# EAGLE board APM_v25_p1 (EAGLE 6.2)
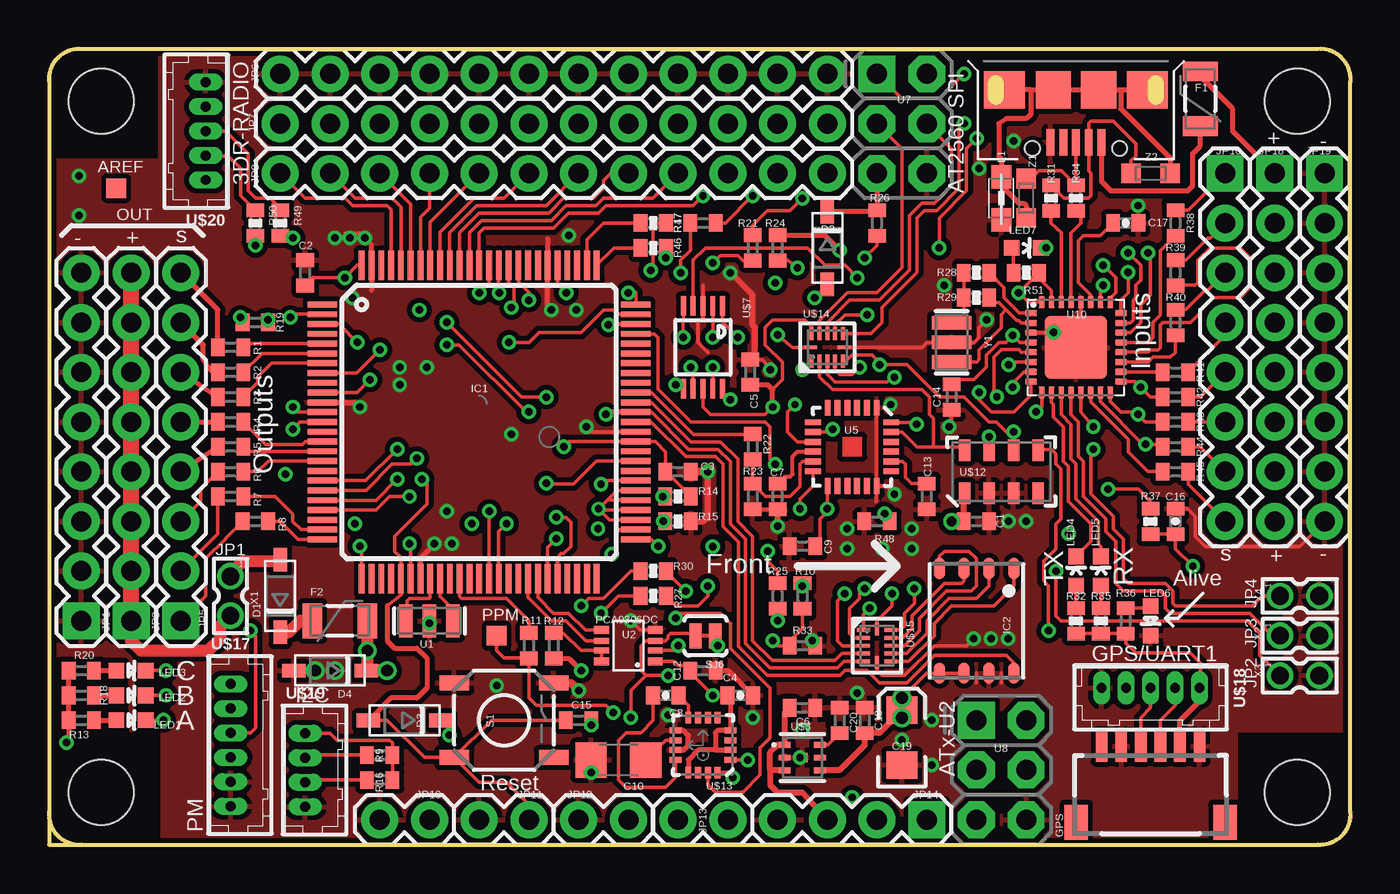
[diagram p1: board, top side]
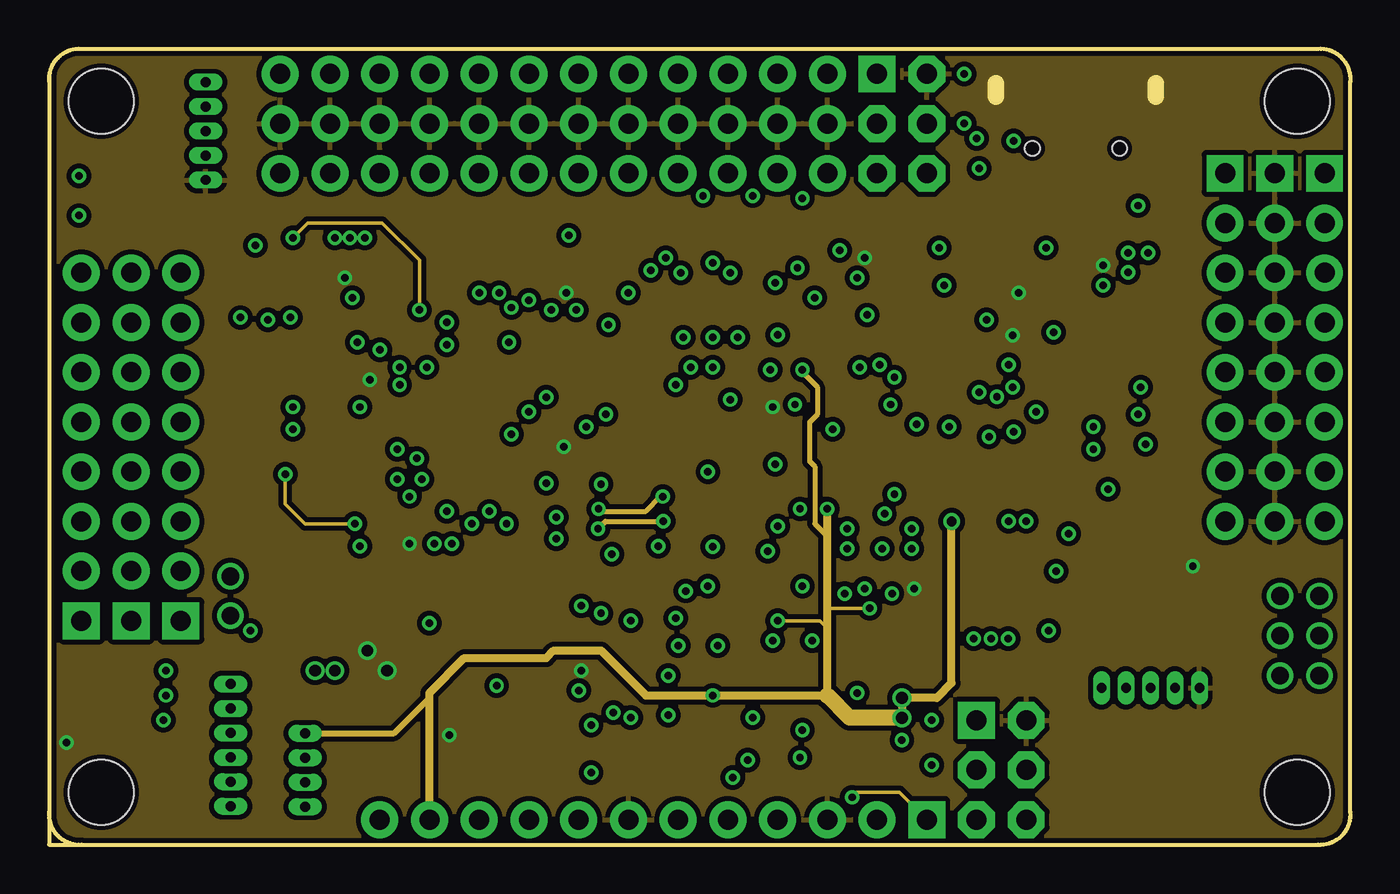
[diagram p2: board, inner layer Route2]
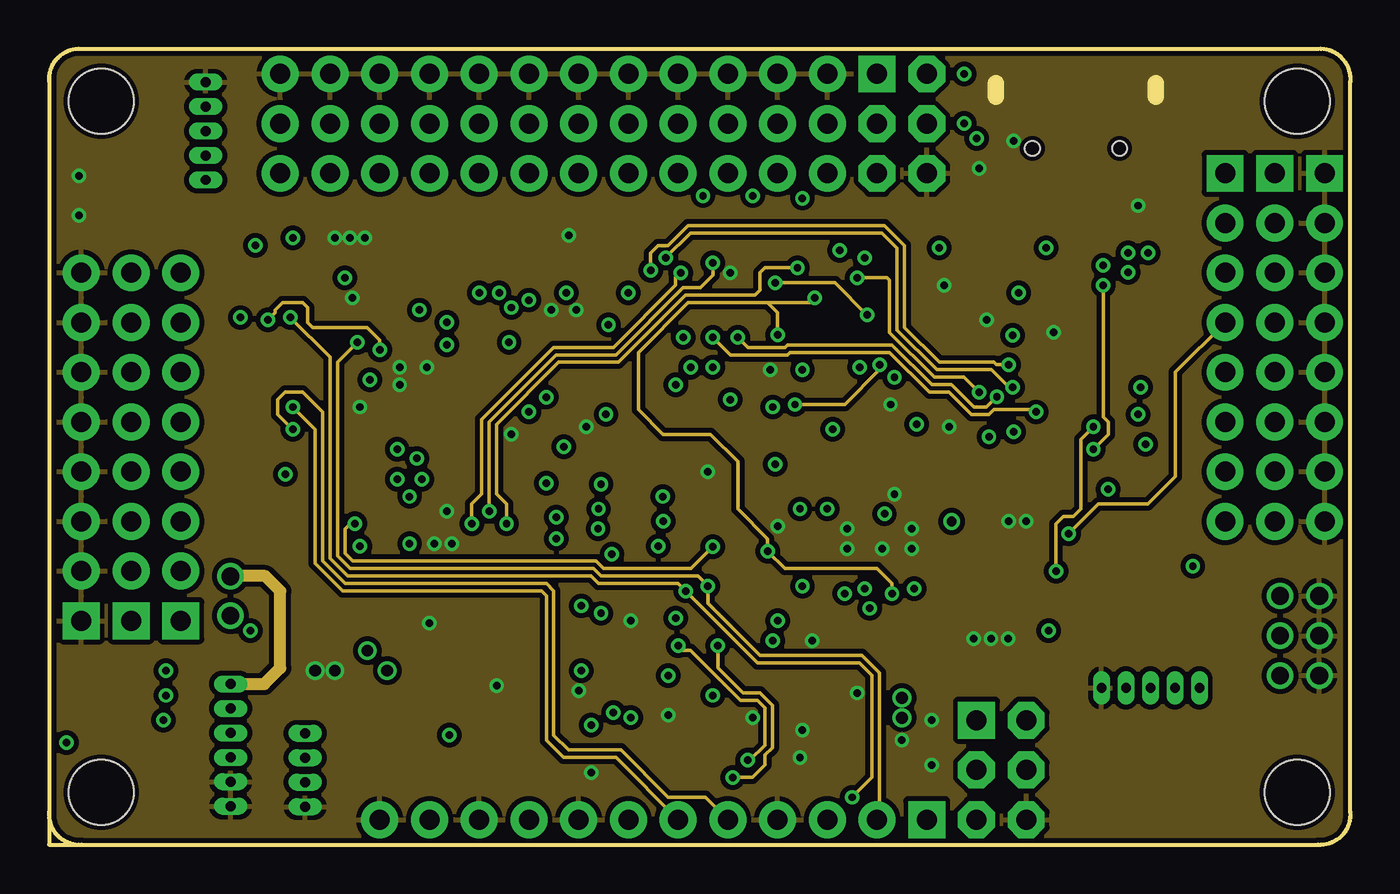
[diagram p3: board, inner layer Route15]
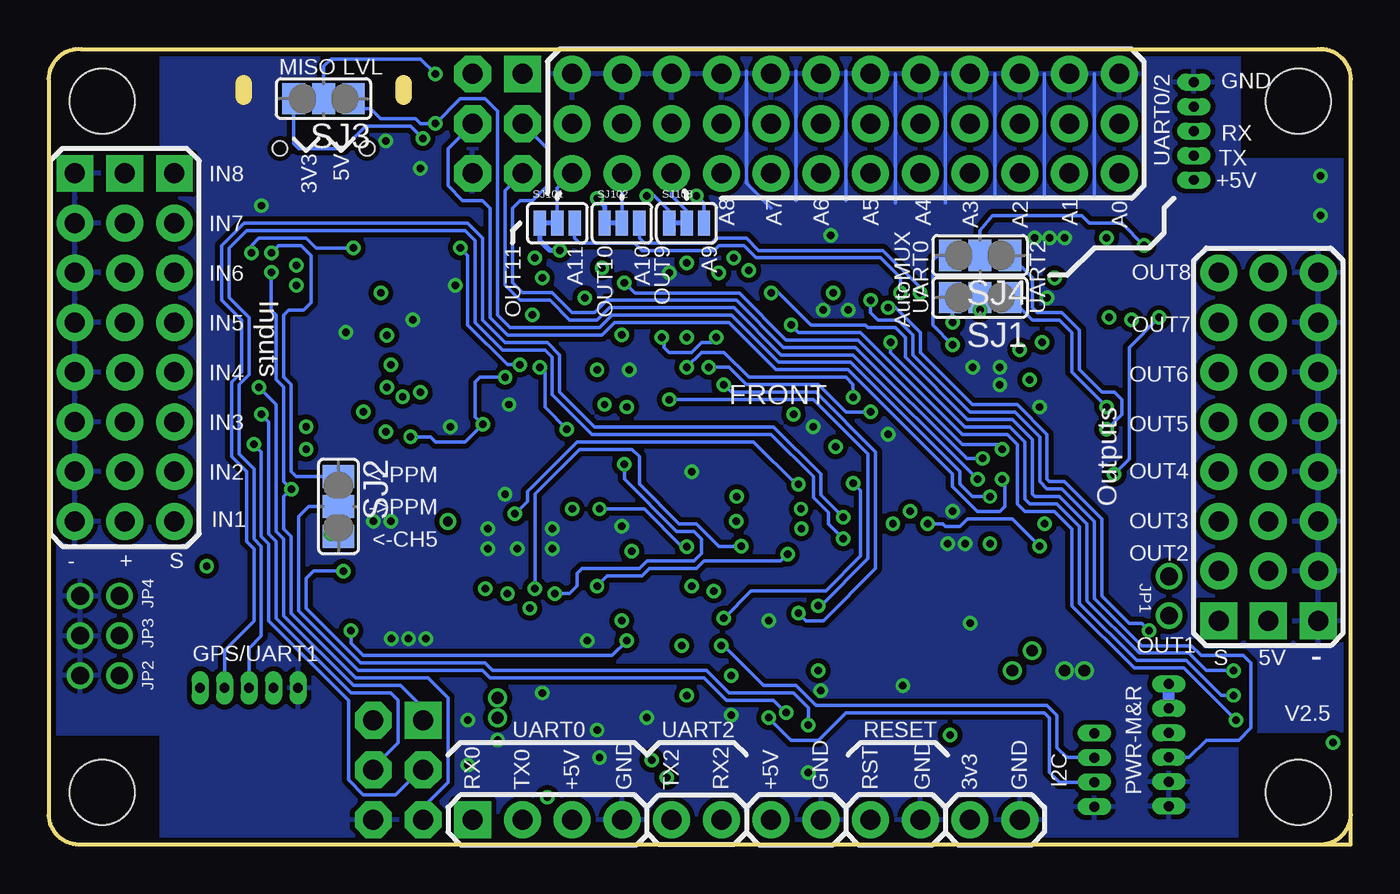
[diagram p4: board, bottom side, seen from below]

Size 66.48 x 40.65 mm. Coordinates in mm from the lower left corner, seen from the top.
Outline: 1.66,0 0,0 0,38.99
Outline: 1.66,0 64.83,0
Outline: 0,39.25 0,38.99
Outline: 1.4,40.64 64.83,40.64 arc-99 66.48,38.98 66.48,1.66 arc-99 64.82,0
Outline: 1.67,40.64 arc99 0,38.99
Outline: 0,1.67 arc99 1.66,0
Copper layers (1*2*15*16): Top 0.035mm / dielectric 0.5mm / Route2 0.035mm / dielectric 0.5mm / Route15 0.035mm / dielectric 0.5mm / Bottom 0.035mm
Design rules: minimum track width 7mil, minimum drill 10mil, track to track 7mil, track to pad 7mil, pad to pad 7mil, via to via 7mil, smd to smd 0mil, copper to edge 10mil, drill to drill 8mil, minimum pad ring 7mil, minimum via ring 7mil, stop-mask expansion 4mil, vias tented up to drill 25mil, thermal gap 10mil
Net classes: 0 default: width 0.178 mm, drill 0.381 mm, clearance 0.178 mm

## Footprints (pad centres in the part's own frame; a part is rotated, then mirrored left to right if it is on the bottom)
C0402 = smd 0.7 x 0.9: 1 -0.65,0; 2 0.65,0
0402-CAP = smd 0.7 x 0.9: 1 -0.65,0; 2 0.65,0
1206 = smd 1.6 x 1.8: 1 -1.4,0; 2 1.4,0
EIA3216 = smd 1.4 x 1.6: A 1.4,0; C -1.4,0
SOD-123 = smd 1.2 x 0.7: A 1.85,0; C -1.85,0
PTC-1206 = smd 1 x 1.8: 1 -1.4,0; 2 1.4,0
SM06B-SRSS-TB = smd 0.6 x 1.55: 1 -2.5,2.975; 2 -1.5,2.975; 3 -0.5,2.975; 4 0.5,2.975; 5 1.5,2.975; 6 2.5,2.975 | smd 1.2 x 1.8: FIT@1 -3.8,-0.9; FIT@2 3.8,-0.9
TQFP100 = smd 1.5 x 0.3: 1 -8,6; 2 -8,5.5; 3 -8,5; 4 -8,4.5; 5 -8,4; 6 -8,3.5; 7 -8,3; 8 -8,2.5; 9 -8,2; 10 -8,1.5; 11 -8,1; 12 -8,0.5; 13 -8,0; 14 -8,-0.5; 15 -8,-1; 16 -8,-1.5; 17 -8,-2; 18 -8,-2.5; 19 -8,-3; 20 -8,-3.5; 21 -8,-4; 22 -8,-4.5; 23 -8,-5; 24 -8,-5.5; 25 -8,-6; 51 8,-6; 52 8,-5.5; 53 8,-5; 54 8,-4.5; 55 8,-4; 56 8,-3.5; 57 8,-3; 58 8,-2.5; 59 8,-2; 60 8,-1.5; 61 8,-1; 62 8,-0.5; 63 8,0; 64 8,0.5; 65 8,1; 66 8,1.5; 67 8,2; 68 8,2.5; 69 8,3; 70 8,3.5; 71 8,4; 72 8,4.5; 73 8,5; 74 8,5.5; 75 8,6 | smd 0.3 x 1.5: 26 -6,-8; 27 -5.5,-8; 28 -5,-8; 29 -4.5,-8; 30 -4,-8; 31 -3.5,-8; 32 -3,-8; 33 -2.5,-8; 34 -2,-8; 35 -1.5,-8; 36 -1,-8; 37 -0.5,-8; 38 0,-8; 39 0.5,-8; 40 1,-8; 41 1.5,-8; 42 2,-8; 43 2.5,-8; 44 3,-8; 45 3.5,-8; 46 4,-8; 47 4.5,-8; 48 5,-8; 49 5.5,-8; 50 6,-8; 76 6,8; 77 5.5,8; 78 5,8; 79 4.5,8; 80 4,8; 81 3.5,8; 82 3,8; 83 2.5,8; 84 2,8; 85 1.5,8; 86 1,8; 87 0.5,8; 88 0,8; 89 -0.5,8; 90 -1,8; 91 -1.5,8; 92 -2,8; 93 -2.5,8; 94 -3,8; 95 -3.5,8; 96 -4,8; 97 -4.5,8; 98 -5,8; 99 -5.5,8; 100 -6,8
VDFN-8-NO-BOTTOM-PAD = smd 1.1 x 0.6: 1 -2.675,1.905; 2 -2.675,0.635; 3 -2.675,-0.635; 4 -2.675,-1.905; 5 2.675,-1.905; 6 2.675,-0.635; 7 2.675,0.635; 8 2.675,1.905
1X08 = drill 1.016 pad 1.88 square: 1 0,0 | drill 1.016 pad 1.88: 2 2.54,0; 3 5.08,0; 4 7.62,0; 5 10.16,0; 6 12.7,0; 7 15.24,0; 8 17.78,0
1X12 = drill 1.016 pad 1.88: 1 0,0; 2 2.54,0; 3 5.08,0; 4 7.62,0; 5 10.16,0; 6 12.7,0; 7 15.24,0; 8 17.78,0; 9 20.32,0; 10 22.86,0; 11 25.4,0; 12 27.94,0
1X02 = drill 1.016 pad 1.88: 1 0,0; 2 2.54,0
1X04 = drill 1.016 pad 1.88 square: 1 0,0 | drill 1.016 pad 1.88: 2 2.54,0; 3 5.08,0; 4 7.62,0
0805 = smd 1.2 x 1: 1 -1.1,0; 2 1.1,0
LED-0603 = smd 0.8 x 0.8: A 0,-0.75; C 0,0.75
0402-RES = smd 0.7 x 0.9: 1 -0.65,0; 2 0.65,0
TACTILE_SWITCH_SMD = smd 1.524 x 0.762: 1 -2.54,1.905; 2 2.54,1.905; 3 -2.54,-1.905; 4 2.54,-1.905
SJ_2 = smd 1.168 x 1.6: 1 -1.524,0; 2 0,0; 3 1.524,0
SJ_2S-TRACE = smd 0.635 x 1.27: 1 -0.508,0; 2 0.508,0
SJ_3 = smd 0.635 x 1.27: 1 -0.889,0; 2 0,0; 3 0.889,0
TP10SQ = smd 1 x 1: TP 0,0
RESONATOR-SMD = smd 0.7 x 1.7: 1 -1.2,0; 2 0,0; 3 1.2,0
VSSOP8 = smd 0.75 x 0.4: 1 -1.375,0.8; 4 -1.375,-0.8; 5 1.375,-0.8; 8 1.375,0.8 | smd 0.75 x 0.3: 2 -1.375,0.25; 3 -1.375,-0.25; 6 1.375,-0.25; 7 1.375,0.25
QFN-24 = smd 0.8 x 0.3: 1 -2,1.25; 2 -2,0.75; 3 -2,0.25; 4 -2,-0.25; 5 -2,-0.75; 6 -2,-1.25; 13 2,-1.25; 14 2,-0.75; 15 2,-0.25; 16 2,0.25; 17 2,0.75; 18 2,1.25 | smd 0.3 x 0.8: 7 -1.25,-2; 8 -0.75,-2; 9 -0.25,-2; 10 0.25,-2; 11 0.75,-2; 12 1.25,-2; 19 1.25,2; 20 0.75,2; 21 0.25,2; 22 -0.25,2; 23 -0.75,2; 24 -1.25,2
2X3-NS = drill 1.016 pad 1.88 square: 1 -2.54,-1.27 | drill 1.016 pad 1.88 octagon: 2 -2.54,1.27; 3 0,-1.27; 4 0,1.27; 5 2.54,-1.27; 6 2.54,1.27
MOLEX_MICRO_USB_AB_BOTTOM_MOUNT = smd 0.4 x 1.35: 1 1.3,-4.125; 2 0.65,-4.125; 3 0,-4.125; 4 -0.65,-4.125; 5 -1.3,-4.125 | smd 2.1 x 1.9: GND1 3.65,-1.452; GND4 -3.65,-1.452 | smd 1.8 x 1.9: GND2 1.151,-1.452; GND3 -1.149,-1.452 | hole 0.75: -2.225,-4.45; 2.225,-4.45
QFN32 = smd 0.6 x 0.3: 1 -2.3,1.75; 2 -2.3,1.25; 3 -2.3,0.75; 4 -2.3,0.25; 5 -2.3,-0.25; 6 -2.3,-0.75; 7 -2.3,-1.25; 8 -2.3,-1.75; 17 2.3,-1.75; 18 2.3,-1.25; 19 2.3,-0.75; 20 2.3,-0.25; 21 2.3,0.25; 22 2.3,0.75; 23 2.3,1.25; 24 2.3,1.75 | smd 0.3 x 0.6: 9 -1.75,-2.3; 10 -1.25,-2.3; 11 -0.75,-2.3; 12 -0.25,-2.3; 13 0.25,-2.3; 14 0.75,-2.3; 15 1.25,-2.3; 16 1.75,-2.3; 25 1.75,2.3; 26 1.25,2.3; 27 0.75,2.3; 28 0.25,2.3; 29 -0.25,2.3; 30 -0.75,2.3; 31 -1.25,2.3; 32 -1.75,2.3 | smd 3.2 x 3.2: EXP 0,0
STAND-OFF = hole 3.302: 0,0
MLF-6 = smd 0.6 x 0.3: 1 -0.9,0.65; 2 -0.9,0; 3 -0.9,-0.65; 4 0.9,-0.65; 5 0.9,0; 6 0.9,0.65 | smd 0.5 x 0.5: 7 0,0
MSOP10 = smd 0.25 x 1: 1 -1,-2.113; 2 -0.5,-2.113; 3 0,-2.113; 4 0.5,-2.113; 5 1,-2.113; 6 1,2.113; 7 0.5,2.113; 8 0,2.113; 9 -0.5,2.113; 10 -1,2.113
MS5611-01BA = smd 1.1 x 0.6: 1 -1.1,1.875; 2 -1.1,0.625; 3 -1.1,-0.625; 4 -1.1,-1.875; 5 1.1,-1.875; 6 1.1,-0.625; 7 1.1,0.625; 8 1.1,1.875
LPCC16 = smd 0.6 x 0.3: 1 -1.4,0.75; 2 -1.4,0.25; 3 -1.4,-0.25; 4 -1.4,-0.75; 9 1.4,-0.75; 10 1.4,-0.25; 11 1.4,0.25; 12 1.4,0.75 | smd 0.3 x 0.6: 5 -0.75,-1.4; 6 -0.25,-1.4; 7 0.25,-1.4; 8 0.75,-1.4; 13 0.75,1.4; 14 0.25,1.4; 15 -0.25,1.4; 16 -0.75,1.4
UQFN-12 = smd 0.2 x 0.65: 1 -0.8,-0.7; 2 -0.4,-0.7; 3 0,-0.7; 4 0.4,-0.7; 5 0.8,-0.7; 7 0.8,0.7; 8 0.4,0.7; 9 0,0.7; 10 -0.4,0.7; 11 -0.8,0.7 | smd 0.65 x 0.2: 6 0.85,0; 12 -0.85,0
DF13-6P-1.25DSA = drill 0.5 pad 0.8 long: 1 -3.125,0; 2 -1.875,0; 3 -0.625,0; 4 0.625,0; 5 1.875,0; 6 3.125,0
DF13-5P-1.25DSA = drill 0.5 pad 0.8 long: 1 -2.5,0; 2 -1.25,0; 3 0,0; 4 1.25,0; 5 2.5,0
DF13-4P-1.25DSA = drill 0.5 pad 0.8 long: 1 -1.875,0; 2 -0.625,0; 3 0.625,0; 4 1.875,0
87758-0216 = drill 0.9 pad 1.27: 1 0,-1; 2 0,1
RESONATOR = smd 0.7 x 2: 1 -1,0; 2 0,0; 3 1,0
CT/CN0603 = smd 1 x 1: 1 -1,0; 2 1,0

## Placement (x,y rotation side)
C1  .1uF  [C0402]  47.38,16.51 180 top
C2  .1uF  [C0402]  13.09,29.21 90 top
C3  .1uF  [C0402]  32.14,19.05 0 top
C4  0.1uF  [0402-CAP]  35.31,7.62 0 top
C5  .1uF  [C0402]  35.82,24.13 270 top
C6  1uF  [C0402]  38.49,6.99 180 top
C7  .1uF  [C0402]  37.22,17.78 90 top
C8  0.22uF  [0402-CAP]  31.5,7.62 180 top
C9  .1uF  [C0402]  38.49,15.24 0 top
C10  4.7uF  [1206]  29.09,4.32 180 top
C12  .1uF  [C0402]  33.41,8.89 180 top
C13  .01uF  [C0402]  44.84,17.78 90 top
C14  .1uF  [C0402]  46.11,22.86 270 top
C15  .1uF  [C0402]  27.06,6.35 180 top
C16  .1uF  [0402-CAP]  57.54,16.51 90 top
C17  1uF  [0402-CAP]  55,31.75 0 top
C18  .01uF  [C0402]  41.66,6.35 270 top
C19  10uf  [EIA3216]  43.57,5.47 90 top
C20  470pF  [C0402]  40.39,6.35 270 top
D1  MBR120VLSFT1G  [SOD-123]  11.82,12.7 90 top
D2  MBR120VLSFT1G  [SOD-123]  39.76,30.48 270 top
D3  MBR120VLSFT1G  [SOD-123]  18.17,6.35 180 top
D4  MMSZ5233BT1G  [SOD-123]  14.36,8.89 180 top
F1  500mA  [PTC-1206]  58.81,38.1 90 top
F2  500mA  [PTC-1206]  14.86,11.43 0 top
GPS  SM06B-SRSS-TB  [SM06B-SRSS-TB]  56.27,2.04 0 top
IC1  ATMEGA2560-16AU  [TQFP100]  21.98,21.59 0 top
IC2  AT45DB161D-MU  [VDFN-8-NO-BOTTOM-PAD]  47.38,11.43 270 top
JP1  GND  [1X08]  1.66,11.43 90 top
JP3  5V  [1X08]  4.2,11.43 90 top
JP5  OUT PWM  [1X08]  6.74,11.43 90 top
JP6  GND  [1X12]  11.82,39.37 0 top
JP7  5V  [1X12]  11.82,36.83 0 top
JP8  IO pins  [1X12]  11.82,34.29 0 top
JP10  3v3  [1X02]  19.44,1.27 180 top
JP11  RST  [1X02]  24.52,1.27 180 top
JP12  VCC  [1X02]  27.06,1.27 0 top
JP13  UART2  [1X02]  34.68,1.27 180 top
JP14  UART0  [1X04]  44.84,1.27 180 top
JP16  IN PWM  [1X08]  60.08,34.29 270 top
JP18  5V  [1X08]  62.62,34.29 270 top
JP19  GND  [1X08]  65.16,34.29 270 top
L1  BLM21  [0805]  48.65,33.02 90 top
LED1  RED  [LED-0603]  4.2,6.35 270 top
LED2  YELLOW  [LED-0603]  4.2,7.62 270 top
LED3  BLUE  [LED-0603]  4.2,8.89 270 top
LED4  ORANGE  [LED-0603]  52.46,13.97 0 top
LED5  ORANGE  [LED-0603]  53.73,13.97 0 top
LED6  GRN  [LED-0603]  56.27,11.43 180 top
LED7  RED  [LED-0603]  49.92,30.48 270 top
R1  220  [C0402]  9.28,25.4 0 top
R2  220  [C0402]  9.28,24.13 0 top
R3  220  [C0402]  9.28,22.86 0 top
R4  220  [C0402]  9.28,21.59 0 top
R5  220  [C0402]  9.28,20.32 0 top
R6  220  [C0402]  9.28,19.05 0 top
R7  220  [C0402]  9.28,17.78 0 top
R8  220  [C0402]  10.55,16.51 0 top
R9  2.2k  [C0402]  16.9,4.58 0 top
R10  4.7K  [C0402]  38.49,12.7 90 top
R11  1K  [C0402]  24.52,10.16 270 top
R12  200k  [C0402]  25.79,10.16 270 top
R13  1k  [C0402]  1.66,6.35 180 top
R14  10K  [0402-RES]  32.14,17.78 180 top
R15  10K  [0402-RES]  32.14,16.51 180 top
R16  2.2k  [C0402]  16.9,3.31 0 top
R17  1k  [C0402]  33.41,31.75 0 top
R18  1k  [C0402]  1.66,7.62 180 top
R19  220  [C0402]  10.55,26.67 0 top
R20  1k  [C0402]  1.66,8.89 180 top
R21  1k  [C0402]  35.95,30.48 90 top
R22  4.7K  [C0402]  35.95,20.32 90 top
R23  10k  [C0402]  35.95,17.78 270 top
R24  1k  [C0402]  37.22,30.48 90 top
R25  10k  [C0402]  37.22,12.7 90 top
R26  10k  [C0402]  42.3,31.75 270 top
R27  1k  [0402-RES]  30.87,12.7 180 top
R28  27  [0402-RES]  47.38,29.21 0 top
R29  1M  [0402-RES]  47.38,27.94 180 top
R30  1k  [0402-RES]  30.87,13.97 180 top
R31  22  [0402-RES]  51.19,33.02 90 top
R32  1k  [0402-RES]  52.46,11.43 90 top
R33  10k  [C0402]  38.49,10.16 0 top
R34  22  [0402-RES]  52.46,33.02 90 top
R35  1k  [0402-RES]  53.73,11.43 90 top
R36  1k  [C0402]  55,11.43 270 top
R37  10K  [0402-RES]  56.27,16.51 270 top
R38  220  [C0402]  57.54,31.75 270 top
R39  220  [C0402]  57.54,29.21 270 top
R40  220  [C0402]  57.54,26.67 270 top
R41  220  [C0402]  57.54,24.13 180 top
R42  220  [C0402]  57.54,22.86 180 top
R43  220  [C0402]  57.54,21.59 180 top
R44  220  [C0402]  57.54,20.32 180 top
R45  220  [C0402]  57.54,19.05 180 top
R46  1k  [0402-RES]  30.87,30.48 0 top
R47  1k  [0402-RES]  30.87,31.75 0 top
R48  10k  [C0402]  42.3,16.51 180 top
R49  1k  [0402-RES]  11.82,31.75 270 top
R50  1k  [0402-RES]  10.55,31.75 270 top
R51  1k  [0402-RES]  49.92,29.21 180 top
S1  [TACTILE_SWITCH_SMD]  23.25,6.35 0 top
SJ1  [SJ_2]  18.93,27.94 180 bottom
SJ2  [SJ_2]  51.69,17.28 270 bottom
SJ3  [SJ_2]  52.46,38.1 180 bottom
SJ4  [SJ_2]  18.93,30.1 180 bottom
SJ6  MAG  [SJ_2S-TRACE]  33.53,10.67 180 top
SJ101  [SJ_3]  40.52,31.75 0 bottom
SJ102  [SJ_3]  37.22,31.75 0 bottom
SJ103  [SJ_3]  33.91,31.75 0 bottom
TP1  TPSQTP10SQ  [TP10SQ]  3.43,33.53 0 top
TP2  TPSQTP10SQ  [TP10SQ]  22.86,10.67 0 top
U1  16MHZ  [RESONATOR-SMD]  19.44,11.43 0 top
U2  PCA9306DC  [VSSOP8]  29.6,10.16 180 top
U5  MPU-6000  [QFN-24]  41.03,20.32 270 top
U7  SPI_Mega  [2X3-NS]  43.57,36.83 270 top
U8  SPI_PPM  [2X3-NS]  48.65,3.81 270 top
U9  USB  [MOLEX_MICRO_USB_AB_BOTTOM_MOUNT]  52.46,40.01 0 top
U10  ATMEGA32U2-MU  [QFN32]  52.46,25.4 0 top
U$1  STAND-OFF  [STAND-OFF]  2.67,37.98 0 top
U$2  STAND-OFF  [STAND-OFF]  2.67,2.67 0 top
U$3  MIC5219-3V3  [MLF-6]  38.49,4.45 0 top
U$4  STAND-OFF  [STAND-OFF]  63.76,37.98 0 top
U$5  STAND-OFF  [STAND-OFF]  63.76,2.67 0 top
U$6  CREATIVE_COMMONS  [CREATIVE_COMMONS]  not placed on the board
U$7  TS5A23157  [MSOP10]  33.41,25.4 180 top
U$12  MS5611-01BA  [MS5611-01BA]  48.65,19.05 90 top
U$13  HMC5883L  [LPCC16]  33.41,5.08 180 top
U$14  TS  [UQFN-12]  39.76,25.4 0 top
U$15  QFN  [UQFN-12]  42.3,10.16 270 top
U$17  DF13-6P-1.25DSA  [DF13-6P-1.25DSA]  9.28,5.08 270 top
U$18  DF13-5P-1.25DSA  [DF13-5P-1.25DSA]  56.27,8.01 180 top
U$19  DF13-4P-1.25DSA  [DF13-4P-1.25DSA]  13.09,3.81 270 top
U$20  DF13-5P-1.25DSA  [DF13-5P-1.25DSA]  8.01,36.45 90 top
X1  ESC 5V EN  [87758-0216]  9.28,12.7 180 top
X2  PPM_PD6  [87758-0216]  63.89,10.67 270 top
X3  HWB  [87758-0216]  63.89,8.64 270 top
X4  PPM_PC4  [87758-0216]  63.89,12.7 270 top
Y1  16MHz  [RESONATOR]  46.11,25.66 90 top
Z1  PGB1010604  [CT/CN0603]  49.92,33.02 270 top
Z2  PGB1010604  [CT/CN0603]  56.27,34.29 0 top

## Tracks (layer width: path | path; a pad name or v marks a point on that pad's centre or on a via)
3.3V  (via drill 0.38, 0.5, 0.6)
  Top 0.178: U2.1 31.92,9.36 32.14,9.15 32.5,9.15 C12.2 32.76,8.78 v33.91,7.62 | U5.13 39.78,17.26 v39.76,17.15 | v39.76,17.15 39.76,17.02 39.37,16.64 39.37,15.5 39.11,15.23 C9.2 | v37.22,11.43 R25.1 | v39.76,17.15 39.74,17.15 | U$14.1 38.93,24.7 v38.49,24.26 | IC2.6 IC2.5 44.83,8.76 v43.57,7.5 | U$15.1 41.6,11.75 v41.91,12.07 | R16.2 R9.2 17.55,5.2 17.4,5.34 14.71,5.34 14.36,5.69 U$19.1
  Top 0.254: v33.91,7.62 C4.1 34.81,7.48 U$13.4 34.16,5.83 34.04,5.72 34.04,4.83 | 34.04,4.83 33.16,4.83 32.66,4.33 U$13.13 | 34.04,4.83 U$13.2
  Top 0.305: U$12.1 46.73,17.91 C1.2 | U$3.4 40.38,3.8 41.66,5.08 C18.2 42.41,5.7 43.18,6.48 v43.57,6.48
  Top 0.406: v43.57,6.48 C19.A | v46.11,16.51 C1.2
  Route2 0.178: v37.22,11.43 39.37,11.43 39.76,11.05 | v41.91,12.07 39.76,12.07
  Route2 0.254: v38.49,24.26 38.49,24.13 39.25,23.37 39.25,21.98 38.87,21.59 38.87,19.56 39.12,19.31 39.12,16.39 39.76,15.75
  Route2 0.305: U$19.1 17.63,5.69 19.44,7.5
  Route2 0.406: JP10.1 19.44,7.5 19.44,7.75 21.21,9.53 25.4,9.53 25.79,9.91 28.2,9.91 30.48,7.62 v33.91,7.62 39.76,7.62 39.76,11.05 39.76,12.07 39.76,15.75 v39.76,17.15 | v43.57,6.48 v43.57,7.5 45.34,7.5 46.11,8.26 v46.11,16.51
  Route2 0.813: v43.57,6.48 40.9,6.48 39.76,7.62
5V
  Top 0.254: 4.32,12.7 4.2,12.83
  Top 0.61: JP3.1 4.2,10.42 4.7,9.91 8.13,9.91 8.77,10.55 8.77,11.2 X1.2
  Top 0.813: JP3.1 4.2,12.83 JP3.2 JP3.3 JP3.4 JP3.5 JP3.6 JP3.7 JP3.8
#RST  (via drill 0.38)
  Top 0.178: U10.13 52.71,22.11 v53.34,21.34 | v51.44,13.97 51.44,11.69 51.69,11.43 61.22,11.43 61.85,10.8 61.85,9.67 X3.1
  Top 0.406: C15.1 27.71,6.12 v27.69,6.1
  Route15 0.178: v53.34,21.34 52.71,20.71 52.71,17.15 52.33,16.77 51.82,16.77 51.44,16.39 v51.44,13.97
  Bottom 0.178: v27.69,6.1 27.69,6.99 28.45,7.75 31.75,7.75 32.9,8.89 43.82,8.89 44.2,9.28 50.55,9.28 53.34,12.07 53.34,13.59 52.96,13.97 v51.44,13.97
CH1
  Top 0.178: R45.1 58.19,18.4 JP16.8
CH5  (via drill 0.38)
  Top 0.178: JP16.4 60.08,26.04 58.19,24.15 R41.1
  Route15 0.178: JP16.4 57.54,24.13 57.54,18.8 56.14,17.4 53.6,17.4 v52.07,15.88
  Bottom 0.178: SJ2.3 52.2,15.75 v52.07,15.88
CH8
  Top 0.178: JP16.1 58.19,32.4 R38.1
CS_DF
  Top 0.178: U$15.9 43.69,10.16 44.45,10.93 44.45,11.56 45.85,12.96 47.12,12.96 47.38,13.21 47.38,14.61 46.99,14.99 45.72,14.99 45.47,14.74 IC2.4
CS_MS5611  (via drill 0.38)
  Top 0.178: U$12.5 50.55,20.18 51.2,20.18 51.44,19.94 51.44,19.44 51.69,19.18 51.69,16.64 51.44,16.39 51.44,15.12 50.8,14.48 50.8,13.47 51.06,13.21 v51.06,10.93 | 38.5,12.07 R10.1 38.49,11.05 37.85,10.42 R33.1 37.22,10.16 v36.96,10.42
  Bottom 0.178: v51.06,10.93 51.06,10.29 50.42,9.66 37.72,9.66 v36.96,10.42
D+
  Top 0.178: Z1.1 50.15,34.02 50.55,34.42 51.71,34.42 R34.2 U9.3
D-
  Top 0.178: R31.2 51.84,33.02 53.09,33.02 53.22,33.15 53.22,34.29 53.11,34.41 U9.2 53.11,36.85 53.22,36.96 54.36,36.96 55.5,35.82 55.5,35.18 55.27,34.95 Z2.1
FSYNC
  Top 0.178: U5.11 38.5,19.57 38.36,19.44 38.36,18.29 37.85,17.78 36.6,17.78 R23.1 R22.1
GND  (via drill 0.38, 0.6)
  Top 0.178: IC1.62 27.69,21.09 v27.44,21.34 | U10.3 v51.32,26.15 | 51.95,25.91 51.71,26.15 v51.32,26.15 | 51.95,25.91 U10.EXP | v51.32,26.15 v51.31,26.17 | U1.2 v19.44,11.31 | U5.1 U5.18 42.77,18.32 v43.18,17.91 | R23.2 C7.1 | C16.2 58.16,17.16 58.55,16.77 58.55,15.75 59.06,15.24 63.89,15.24 JP19.8 | C5.1 36.44,24.78 v36.83,24.26 | U$7.3 33.41,26.93 33.15,26.67 33.15,25.66 33.66,25.15 | 16.48,30.65 v16.13,30.99 15.88,31.25 15.12,31.25 | C14.2 46.11,21.59 v45.98,21.34 | U2.4 30.19,10.96 v29.72,11.43 | U$15.6 42.3,8.89 42.55,8.64 43.69,8.64 45.22,10.16 46.87,10.16 47.25,10.55 | U$14.6 44.58,25.4 44.84,25.66 Y1.2 47.25,25.66 47.5,25.91 47.5,26.42 v47.88,26.8 47.76,26.67 | R33.2 39.14,10.28 v38.99,10.42 | U10.28 52.71,26.67 51.95,25.91 | 33.41,27.69 33.41,28.58 | 47.38,8.77 47.38,8.26 | 48.65,8.77 48.65,8.26 | 42.27,18.24 42.27,17.56 42.24,17.53
  Top 0.254: IC1.11 15.61,22.59 v15.88,22.36 | IC1.81 25.48,27.49 v25.66,27.31 | IC1.62 | 16.48,30.65 IC1.99 16.48,28.32 | C4.2 34.68,8.89 C12.1 | U$13.11 32.39,4.83 32.64,5.08 32.64,5.59 32.4,5.83 U$13.9 | IC1.32 18.98,14.66 v19.69,15.37 | IC1.81 25.48,30.94
  Top 0.305: C7.1 v37.22,16.26 | R15.1 33.41,16.51 33.66,16.77 v33.66,19.05 | v34.8,29.21 35.95,28.07 35.95,26.55 36.07,26.42 36.07,25.04 C5.1
  Top 0.406: C3.2 33.14,19.04 v33.66,19.05 | S1.2 26.67,8.26 v27.06,7.88
  Bottom 0.178: 13.09,33.02 13.09,39.37 | 15.63,33.02 15.63,39.37 | 18.17,33.02 18.17,39.37 | 20.71,32.77 20.71,39.37 | 23.25,32.77 23.25,39.37 | 25.79,32.9 25.79,39.5 | 28.33,32.9 28.33,39.5 | 30.87,39.5 30.87,33.79 29.6,32.52
  other vias: 19.31,24.39 22.86,8.13 23.63,20.96 47.5,34.55 45.72,28.58 17.91,24.39 17.91,23.5 20.32,17.02 15.5,27.94 27.69,3.69 45.09,4.07 1.53,32.14 1.53,34.17 45.09,6.35 49.03,16.51 43.57,5.34 38.36,4.45 31.63,6.61 35.95,6.48 38.49,5.85 41.28,7.75 49.28,35.95 55.63,32.64 13.59,8.89 14.61,8.89 49.92,16.51 44.07,16.13 44.07,15.12 42.55,15.12 40.77,15.12 40.77,16.13 42.98,22.48 15.37,30.99 14.61,30.99 20.58,15.37 26.93,27.31 26.55,31.12 48.11,10.52 49,10.52 47.22,10.52
  pour Top (isolate 0.254): 14.74,28.96 29.21,28.83 29.21,14.23 14.74,14.36
  pour Bottom (isolate 0.254): 5.72,40.64 60.71,40.64 60.71,35.06 70.24,35.06 70.24,5.72 60.71,5.72 60.71,0 5.85,0 5.85,5.85 0,5.85 0,34.93 5.72,34.93
  pour Route15 (isolate 0.254): 0,40.64 67.7,40.64 67.7,0 0,0
  pour Top (isolate 0.254): 0,34.93 5.72,34.93 5.72,40.64 60.71,40.64 60.71,35.06 71.51,35.06 71.51,5.85 60.58,5.85 60.58,0 5.85,0 5.85,5.85 0,5.85
HI  (via drill 0.38)
  Top 0.178: IC1.54 28.13,17.09 v28.07,17.15 | IC1.55 29.96,17.61 28.53,17.61 v28.07,17.15 | IC1.53 28.63,16.59 v28.07,17.15 | IC1.56 29.02,18.09 v28.07,17.15
  Top 0.254: v31.36,17.78 R14.2
  Route2 0.254: v31.36,17.78 31.25,17.78 30.48,17.02 28.2,17.02 v28.07,17.15
IN0
  Top 0.178: 53.21,22.62 U10.14 53.22,23.09 53.22,22.61 55.12,20.71 55.12,20.07 56.14,19.05 R45.2
IN4
  Top 0.178: U10.18 56.87,24.15 R41.2
IN5
  Top 0.178: R40.2 57.54,25.15 57.28,24.9 56.39,24.9 56.15,24.65 U10.19
IN6
  Top 0.178: 57.52,28.58 R39.2 57.55,28.58 58.55,28.58 58.68,28.71 58.68,29.85 59.31,30.48 60.84,30.48 61.35,29.98 61.35,28.45 60.84,27.94 59.44,27.94 58.81,27.31 58.81,27.18 58.3,26.67 56.9,26.67 56.77,26.55 56.77,25.4 56.65,25.28 56.27,25.28 56.14,25.15 U10.20
IN7
  Top 0.178: U10.21 56.13,25.65 56.39,25.91 56.39,26.67 56.77,27.06 56.77,30.34 R38.2
INT  (via drill 0.38)
  Top 0.178: v38.36,17.15 38.36,17.66 39.03,18.33 U5.12 | R19.1 9.9,26.82 v9.78,26.93
  Route2 0.178: v12.07,18.93 12.07,17.4 13.09,16.39 v15.63,16.39
  Route15 0.178: v33.91,15.23 32.79,14.1 28.33,14.1 27.94,14.48 15.5,14.48 15.12,14.86 15.12,16.13 15.37,16.39 v15.63,16.39
  Bottom 0.178: v38.36,17.15 36.07,17.15 34.17,15.24 v33.91,15.23 | v9.78,26.93 11.31,25.4 11.31,19.69 v12.07,18.93
JP_RX  (via drill 0.38)
  Top 0.178: v12.45,30.99 11.93,30.99 R49.2
  Route2 0.178: v18.93,27.31 18.93,29.85 17.02,31.75 13.21,31.75 v12.45,30.99
  Bottom 0.178: SJ1.2 v18.93,27.31
JP_TX  (via drill 0.38)
  Top 0.178: v10.55,30.61 R50.2
  Bottom 0.178: v10.55,30.61 11.69,31.75 13.34,31.75 13.72,32.14 18.29,32.14 18.93,31.37 SJ4.2
JP_VCC
  Top 0.406: 11.76,14.61 D1.A
  Top 0.61: X1.1 9.28,13.85 9.91,14.48 11.74,14.48 D1.A
  Route15 0.61: U$17.1 11,8.21 11.82,9.02 11.82,12.96 11.05,13.72 9.29,13.72 X1.1
  Bottom 0.61: U$17.2 U$17.1
LO  (via drill 0.38)
  Top 0.254: v31.37,16.51 R15.2
  Route2 0.254: v28.05,16.13 28.43,16.51 v31.37,16.51
MISO_3V3  (via drill 0.38)
  Top 0.178: 49.27,21.08 U$12.6 | v49.28,21.09 49.27,21.08 | U5.9 38.24,20.57 37.72,21.09 37.72,22.1 v38.1,22.48 | U$14.5 40.71,24.7 41.03,25.02 42.04,25.02 42.42,24.64 v42.42,24.52 43.82,24.52 45.47,22.86 46.74,22.86 48.01,21.59 48.39,21.59 48.91,21.08 49.27,21.08 | v45.47,30.48 45.47,32.01 46.87,33.41 46.87,35.56 v47.38,36.07
  Route15 0.178: v38.1,22.48 40.64,22.48 42.42,24.26 v42.42,24.52
  Bottom 0.178: v42.42,24.52 43.06,24.52 45.09,26.55 45.09,30.1 v45.47,30.48 | v47.38,36.07 48.01,36.71 50.3,36.71 51.44,35.56 53.73,35.56 53.98,35.82 SJ3.3
MOSI_3V3  (via drill 0.38)
  Top 0.178: U$12.7 48.02,20.82 v48.01,20.83 | U5.24 44.22,21.57 v44.33,21.47 | U$14.3 39.76,24.01 40.14,23.63 42.8,23.63 v43.18,23.88
  Bottom 0.178: v48.01,20.83 46.99,20.83 46.74,20.58 45.22,20.58 v44.33,21.47 44.71,21.85 44.71,23.63 44.45,23.88 v43.18,23.88
MOSI_DF
  Top 0.178: U$15.7 43.91,9.36 45.22,10.67 45.22,11.31 46.11,12.2 48.26,12.2 49.28,13.21 IC2.1
MUX_RX  (via drill 0.38)
  Top 0.178: U$7.9 v33.91,24.38 v33.91,24.39 | v25.4,22.86 24.13,22.86 v20.32,26.67
  Bottom 0.178: v33.91,24.39 33.15,25.15 32.01,25.15 30.74,23.88 25.79,23.88 25.4,23.5 v25.4,22.86 | v20.32,26.67 20.32,27.82 SJ1.3
MUX_TX  (via drill 0.38)
  Top 0.178: U$7.7 32.91,24.25 v32.77,24.39 | v24.52,22.1 24.39,22.1 20.96,25.53 v20.32,25.53
  Bottom 0.178: v32.77,24.39 31.75,24.39 30.87,23.5 27.18,23.5 25.79,22.1 v24.52,22.1 | v20.32,25.53 21.34,26.55 21.34,29.85 21.09,30.1 SJ4.3 19.05,30.1
N$1
  Top 0.178: R36.1 56.17,12.08 LED6.A
N$2
  Top 0.178: U5.20 43.6,19.57 43.74,19.44 43.74,18.75 44.05,18.44 C13.2
N$3
  Top 0.203: U5.10 38.24,20.07 37.98,19.82 37.98,18.93 37.85,18.8 37.59,18.8 C7.2
N$4
  Top 0.178: U$3.6 39.79,5.1 C20.2
N$5
  Top 0.61: D1.C 12.25,10.85 12.83,11.43 F2.1
N$7
  Top 0.178: U$13.10 31.5,5.33 C10.1
N$8
  Top 0.254: JP5.5 R4.1
N$9
  Top 0.254: JP5.6 R3.1
N$10
  Top 0.254: JP5.7 7.88,25.53 7.88,24.77 8.01,24.64 8.01,24.52 8.39,24.13 R2.1
N$11
  Top 0.254: R1.1 8.63,27.32 JP5.8
N$12
  Top 0.178: U2.8 U2.7 27.18,9.91 26.29,10.8 25.8,10.8 R12.1
N$13
  Top 0.254: JP5.4 R5.1
N$14
  Top 0.178: R6.1 8.63,19.04 7.75,18.17 7.75,17.53 JP5.3
N$15
  Top 0.178: R7.1 8.63,15.86 JP5.2
N$16
  Top 0.178: R8.1 9.02,15.64 9.02,15.63 8.01,14.61 8.01,12.7 JP5.1
N$17
  Bottom 0.178: 19.05,27.94 20.32,27.94
N$18
  Top 0.178: R51.2 49.27,30.38 LED7.A
N$19
  Top 0.178: JP16.2 59.31,30.99 59.19,30.99 58.06,29.86 R39.1
N$20
  Top 0.178: R40.1 58.06,27.32 59.06,28.33 59.19,28.33 JP16.3
N$21
  Bottom 0.178: 51.19,38.23 52.2,38.23
N$22
  Top 0.178: R42.1 58.81,22.86 JP16.5
N$23
  Top 0.178: R43.1 JP16.6
N$24
  Top 0.178: R44.1 58.81,20.32 JP16.7
N$25  (via drill 0.38)
  Top 0.178: U$13.16 34.68,3.68 v34.93,3.43 | v34.17,10.16 SJ6.1
  Route15 0.178: v34.93,3.43 35.95,3.43 36.58,4.07 36.58,4.58 36.96,4.96 36.96,7.12 36.33,7.75 35.44,7.75 34.17,9.02 v34.17,10.16
N$26
  Top 0.178: U$13.8 32.66,7.12 C8.1
N$27
  Top 0.178: C8.2 30.85,6.34 30.23,5.72 29.47,5.72 29.09,5.34 29.09,3.31 29.47,2.93 31.5,2.93 32.01,3.43 U$13.12
N$28
  Top 0.254: R13.1 LED1.A
N$29
  Top 0.178: LED5.A R35.2
N$30
  Top 0.178: LED4.A R32.2
N$31
  Top 0.254: R18.1 LED2.A
N$32  (via drill 0.38)
  Top 0.178: R30.2 29.72,13.97 28.33,12.58 27.56,12.58 v27.18,12.2 | U$7.10 34.41,23.1 v34.8,22.74
  Bottom 0.178: v27.18,12.2 27.06,12.2 24.64,14.61 24.64,19.94 27.44,22.74 v34.8,22.74
N$33  (via drill 0.38)
  Top 0.178: R27.2 29.09,12.7 v28.2,11.82 | U$7.6 32.41,23.39 32.37,23.39 32.26,23.5 v32.01,23.5
  Bottom 0.178: v28.2,11.82 27.82,11.43 26.93,11.43 24.26,14.1 24.26,20.07 27.31,23.12 31.63,23.12 v32.01,23.5
N$34
  Top 0.254: R20.1 LED3.A
N$36  (via drill 0.38)
  Top 0.178: R17.2 34.55,31.75 v35.95,33.15
  Bottom 0.178: v35.95,33.15 35.56,33.15 34.8,32.39 SJ103.1
N$38  (via drill 0.38)
  Top 0.254: R24.2 39.61,31.13 v40.39,30.36
  Bottom 0.254: v40.39,30.36 40.9,30.36 41.41,30.87 SJ101.1
N$39  (via drill 0.38)
  Top 0.178: R21.2 35.95,31.63 36.71,32.39 37.85,32.39 v38.49,33.02
  Bottom 0.254: v38.49,33.02 38.23,32.77 38.1,32.64 SJ102.1
N$40
  Bottom 0.254: 34.04,31.75 34.68,31.75
N$41
  Bottom 0.254: 37.34,31.75 37.98,31.75
N$42
  Bottom 0.254: 40.77,31.75 41.15,31.75
N$56
  Top 0.178: IC1.34 19.98,12.67 20.64,12.01 U1.3 20.58,11.49
N$89
  Top 0.178: IC1.33 19.48,12.62 19.44,12.58 18.42,12.58 18.29,12.45 18.29,11.49 U1.1
PA1
  Top 0.178: IC1.77 27.48,30.9 28.33,31.75 R47.1
PA2
  Top 0.178: R46.1 28.87,30.48 IC1.76
PA3  (via drill 0.38)
  Top 0.178: IC1.75 29.98,28.2 v29.6,28.2 | LED3.C v5.97,8.89
  Bottom 0.178: v29.6,28.2 29.21,28.2 27.56,26.55 24.77,26.55 24.64,26.42 23.25,26.42 22.74,25.91 22.74,24.9 19.56,21.72 17.28,21.72 16.26,20.71 16.26,17.91 16.13,17.78 14.86,17.78 13.47,16.39 13.47,12.45 10.8,9.78 8.26,9.78 7.37,8.89 v5.97,8.89
PA4  (via drill 0.38)
  Top 0.178: IC1.74 29.05,27.09 28.83,27.31 28.33,27.31 27.18,26.17 25.02,26.17 24.52,25.66 v23.5,25.66 | LED2.C v5.97,7.62
  Bottom 0.178: v23.5,25.66 23.5,25.15 19.69,21.34 17.4,21.34 16.64,20.58 16.64,17.66 16.39,17.4 14.99,17.4 13.85,16.26 13.85,12.32 10.93,9.4 8.39,9.4 6.61,7.62 v5.97,7.62
PA5  (via drill 0.38)
  Top 0.178: IC1.73 28.63,26.59 v28.58,26.55 | LED1.C v5.85,6.35
  Bottom 0.178: v28.58,26.55 28.2,26.17 25.02,26.17 19.82,20.96 17.53,20.96 17.02,20.45 17.02,17.4 16.64,17.02 15.12,17.02 14.23,16.13 14.23,12.2 11.05,9.02 8.51,9.02 v5.85,6.35
PA6  (via drill 0.38)
  Top 0.178: IC1.72 30.94,26.09 31.12,25.91 31.12,23.27 32.8,21.59 36.58,21.59 36.83,21.34 36.83,19.69 v37.09,19.44 | U$15.3 40.52,10.16 40.26,10.42 40.26,12.45 v40.64,12.83
  Bottom 0.178: v37.09,19.44 37.09,18.67 34.42,16.01 33.53,16.01 33.15,15.63 33.15,14.86 33.53,14.48 35.95,14.48 36.33,14.1 39.25,14.1 39.5,13.85 39.5,13.21 39.88,12.83 v40.64,12.83
PB0  (via drill 0.38)
  Top 0.178: IC1.19 16.18,18.59 v17.78,20.2 | U$14.8 40.16,26.57 40.64,27.06 v41.79,27.06
  Route15 0.178: v41.79,27.06 40.14,28.71 v37.09,28.71
  Bottom 0.178: v37.09,28.71 36.56,28.17 31.22,28.17 28.83,25.79 25.15,25.79 19.82,20.45 18.04,20.45 v17.78,20.2
PB1  (via drill 0.38)
  Top 0.178: IC1.20 16.19,18.09 17.53,19.44 18.51,19.44 v18.8,19.73 | U$14.10 39.36,26.78 40.77,28.2 42.3,28.2 43.57,29.47 43.57,35.56 U7.3
  Bottom 0.178: U7.3 41.03,35.56 41.03,33.66 41.79,32.9 42.42,32.9 42.8,32.52 42.8,28.71 42.3,28.2 40.77,28.2 39.76,27.18 38.61,27.18 37.98,27.82 31.37,27.82 28.96,25.4 25.28,25.4 19.6,19.73 v18.8,19.73
PB2  (via drill 0.38)
  Top 0.178: IC1.21 16.71,17.59 v17.78,18.67 | U$14.9 39.76,26.67 40.9,27.82 42.42,27.82 43.95,29.34 43.95,32.14 44.58,32.77 45.22,32.77 46.11,33.66 46.11,35.56 U7.4
  Bottom 0.178: U7.4 46.11,35.56 46.11,33.66 45.34,32.9 44.33,32.9 43.95,32.52 43.95,26.93 43.06,26.04 38.23,26.04 37.6,26.67 31.75,26.67 29.34,24.26 25.66,24.26 20.32,18.93 20.32,18.29 19.05,17.02 17.91,17.02 17.66,17.28 17.66,18.55 v17.78,18.67
PB3  (via drill 0.38)
  Top 0.178: v18.42,17.78 17.4,17.78 16.71,17.09 IC1.22 | U$14.7 41.98,26.1 42.55,26.67 42.55,27.44 44.33,29.21 44.33,32.01 44.71,32.39 45.34,32.39 46.49,33.53 46.49,36.58 v46.74,36.83
  Bottom 0.178: v18.42,17.78 19.31,17.78 19.94,18.42 19.94,19.05 25.53,24.64 29.21,24.64 31.63,27.06 37.72,27.06 38.36,26.42 42.93,26.42 43.57,27.06 43.57,37.47 44.2,38.1 45.47,38.1 v46.74,36.83 47.5,36.83 47.76,37.09 49.53,37.09 50.04,37.6 50.42,37.6 SJ3.1
PB3_PIN  (via drill 0.38)
  Top 0.178: U7.1 43.57,38.1 45.47,38.1 v46.74,39.37
  Bottom 0.178: SJ3.2 52.46,39.76 52.07,40.14 47.5,40.14 v46.74,39.37
PB5
  Top 0.178: IC1.24 12.87,16.09 12.45,16.51 12.45,16.9 11.56,17.78 R7.2
PB6
  Top 0.178: IC1.25 12.74,15.59 11.82,16.51 R8.2
PB7  (via drill 0.38)
  Top 0.178: 32.52,31.75 R17.1 32.77,31.74 32.77,30.36 32.26,29.85 v32.26,29.21 | IC1.26 15.98,15.15 v15.88,15.24
  Route15 0.178: v21.59,16.39 21.59,17.4 22.1,17.91 22.1,21.72 25.79,25.4 28.83,25.4 32.01,28.58 32.01,28.96 v32.26,29.21
  Bottom 0.178: v21.59,16.39 20.83,16.39 20.71,16.26 19.94,16.26 19.56,16.64 17.28,16.64 v15.88,15.24
PC4  (via drill 0.38)
  Top 0.178: IC1.57 28.37,18.59 v28.2,18.42 | R48.1 42.66,16.91 v42.68,16.9
  Bottom 0.178: v28.2,18.42 28.33,18.42 30.48,20.58 39.5,20.58 42.04,18.04 42.04,17.53 v42.68,16.9
PC6  (via drill 0.38)
  Top 0.178: U$13.15 33.66,3.06 34.04,2.67 35.44,2.67 36.33,3.56 36.33,4.96 36.83,5.47 36.83,8.01 34.8,10.04 34.8,11.31 34.29,11.82 32.26,11.82 v32.01,11.56 | IC1.59 27.98,19.59 26.8,18.42 25.46,18.42 v25.4,18.47
  Bottom 0.178: v32.01,11.56 30.61,12.96 26.8,12.96 25.02,14.74 25.02,18.09 v25.4,18.47
PC7_LED  (via drill 0.38)
  Top 0.178: LED7.C v50.93,30.48 | U10.22 55.24,26.15 55.76,26.67 55.76,27.56 56.27,28.07 56.27,30.1 v56.14,30.23
  Bottom 0.178: v50.93,30.48 52.84,30.48 53.34,30.99 55.76,30.99 56.14,30.61 v56.14,30.23
PD0
  Top 0.178: U2.6 27.44,10.42 26.42,11.43 25.66,11.43 24.48,12.62 IC1.43
PD1
  Top 0.178: U2.5 27.4,10.96 26.55,11.82 25.79,11.82 24.98,12.63 IC1.44
PD2  (via drill 0.38)
  Top 0.178: IC1.45 25.48,15.19 v25.91,15.63 | GPS.3 55.77,6.49 56.27,6.99 U$18.3
  Bottom 0.178: v25.91,15.63 26.67,16.39 26.67,16.97 27.44,17.73 27.44,18.8 29.6,20.96 38.74,20.96 40.77,22.99 40.77,24.9 41.15,25.28 43.31,25.28 44.71,26.67 44.71,30.87 45.22,31.37 56.39,31.37 57.28,30.48 57.28,27.94 56.27,26.93 56.27,24.01 56.77,23.5 56.77,19.94 56.01,19.18 56.01,15.63 55.63,15.24 55.63,10.67 56.27,10.04 U$18.3
PD3  (via drill 0.38)
  Top 0.178: IC1.46 25.98,14.67 26.17,14.86 26.29,14.86 26.67,15.24 26.67,16.46 26.42,16.72 v25.91,16.72 | GPS.4 56.77,6.35 57.54,7.12 57.54,7.99 U$18.2
  Bottom 0.178: v25.91,16.72 27.06,17.86 27.06,18.93 29.47,21.34 38.61,21.34 40.39,23.12 40.39,25.02 41.03,25.66 43.18,25.66 44.33,26.8 44.33,30.99 45.09,31.75 56.52,31.75 57.66,30.61 57.66,27.82 56.65,26.8 56.65,24.13 57.15,23.63 57.15,19.82 56.39,19.05 56.39,15.5 56.01,15.12 56.01,11.43 57.52,9.93 U$18.2
PE0  (via drill 0.38)
  Top 0.178: IC1.2 12.49,27.09 v12.32,26.93 | R30.1 31.52,13.96 v32.52,12.96
  Route2 0.178: v41.03,2.42 41.28,2.67 43.44,2.67 JP14.1
  Route15 0.178: v12.32,26.93 14.36,24.9 14.36,14.61 15.24,13.72 27.69,13.72 28.07,13.34 32.14,13.34 v32.52,12.96 36.2,9.28 41.41,9.28 42.04,8.64 42.04,3.43 v41.03,2.42
PE1  (via drill 0.38)
  Top 0.178: IC1.3 14.82,26.59 v15.75,25.66 | v33.66,13.21 33.66,12.7 33.15,12.2 32.02,12.2 R27.1
  Route15 0.178: v15.75,25.66 14.74,24.64 14.74,14.74 15.37,14.1 27.82,14.1 28.2,13.72 33.15,13.72 v33.66,13.21 33.66,12.32 36.33,9.66 41.53,9.66 42.42,8.77 42.42,1.4 JP14.2
PE3
  Top 0.178: IC1.5 10.12,25.59 R1.2
PE4
  Top 0.178: IC1.6 10.89,25.09 R2.2
PE5
  Top 0.178: IC1.7 11.39,24.59 10.67,23.88 10.67,23.61 R3.2
PE6  (via drill 0.38)
  Top 0.178: IC1.8 15.71,24.09 v16.9,25.28 | R19.2 11.2,26.79 v11.18,26.8
  Route15 0.178: v16.9,25.28 16.9,25.79 16.26,26.42 13.47,26.42 13.21,26.67 13.21,27.44 12.96,27.69 11.94,27.69 11.56,27.31 11.56,27.18 v11.18,26.8
PF0
  Top 0.178: IC1.97 17.48,32.44 17.28,32.64 15.5,32.64 15.12,33.02 13.09,33.02 JP8.1
PF1
  Top 0.178: IC1.96 17.98,32.58 17.53,33.02 15.63,33.02 JP8.2
PF2
  Top 0.178: IC1.95 18.48,32.71 JP8.3
PF3
  Top 0.178: IC1.94 18.98,32.06 19.44,32.52 JP8.4
PF4
  Top 0.178: IC1.93 19.48,31.79 JP8.5
PF5
  Top 0.178: IC1.92 19.98,31.28 21.72,33.02 23.25,33.02 JP8.6
PF6
  Top 0.178: IC1.91 20.48,31.27 21.85,32.64 25.4,32.64 JP8.7
PF7
  Top 0.178: IC1.90 20.98,31.26 21.98,32.26 25.53,32.26 26.29,33.02 27.82,33.02 28.33,33.53 28.33,33.91 28.71,34.29 JP8.8
PG0  (via drill 0.38)
  Top 0.178: IC1.51 30.77,15.59 v31.12,15.24 | U$15.2 41.13,10.56 40.9,10.8 40.9,12.07 41.41,12.58 41.41,12.83 v41.66,13.09
  Bottom 0.178: v31.12,15.24 32.26,15.24 33.41,16.39 34.29,16.39 36.33,18.42 36.33,19.82 36.71,20.2 39.37,20.2 41.66,17.91 v41.66,13.09
PG1  (via drill 0.38)
  Top 0.178: IC1.52 29.18,16.09 28.94,15.85 28.94,15.02 v28.76,14.84 | v38.49,13.21 R10.2
  Route2 0.178: v28.76,14.84 28.76,14.86
  Bottom 0.178: v38.49,13.21 37.98,13.72 36.2,13.72 35.82,14.1 33.41,14.1 33.02,14.48 29.11,14.48 v28.76,14.84
PH0  (via drill 0.38)
  Top 0.178: IC1.12 12.7,22.09 v12.45,22.36
  Route15 0.178: v12.45,22.36 13.59,21.21 13.59,14.36 14.99,12.96 25.15,12.96 25.4,12.7 25.4,5.34 26.29,4.45 28.96,4.45 JP13.2
  Bottom 0.178: v12.45,22.36 14.23,24.13 14.23,26.17 14.86,26.8 16.26,26.8 SJ1.1
PH1  (via drill 0.38)
  Top 0.178: IC1.13 12.83,21.59 v12.45,21.21
  Route15 0.178: v12.45,21.21 11.69,21.98 11.69,22.74 12.07,23.12 12.96,23.12 13.97,22.1 13.97,14.48 15.12,13.34 25.4,13.34 25.79,12.96 25.79,5.59 26.55,4.83 29.21,4.83 31.63,2.42 33.53,2.42 JP13.1
  Bottom 0.178: v12.45,21.21 11.69,21.98 11.69,22.74 12.07,23.12 12.7,23.12 13.85,24.26 13.85,26.29 14.74,27.18 16.01,27.18 16.26,27.44 16.26,28.96 SJ4.1
PH3
  Top 0.178: IC1.15 13.1,20.59 12.96,20.45 11.07,20.45 R4.2
PH4
  Top 0.178: IC1.16 10.2,20.09 R5.2
PH5
  Top 0.178: IC1.17 11.21,19.59 10.67,19.05 R6.2
PJ0
  Top 0.178: IC1.63 30.76,21.59 32.54,19.82 34.04,19.82 34.42,19.44 34.42,16.26 35.21,15.47 35.21,10.14 36.71,8.64 40.39,8.64 40.64,8.89 41.79,8.89 42.42,8.26 43.82,8.26 45.22,9.66 48.9,9.66 49.28,9.28 IC2.8
PJ1  (via drill 0.38)
  Top 0.178: IC1.64 30.77,22.09 32.67,20.2 34.17,20.2 34.8,19.56 34.8,16.39 35.56,15.63 35.56,10.29 36.83,9.02 40.26,9.02 40.61,9.36 U$15.5
  Top 0.254: IC1.64 28.59,22.09 v28.45,21.98
PJ2
  Top 0.178: IC1.65 30.78,22.59 32.8,20.58 34.29,20.58 35.18,19.69 35.18,16.51 35.95,15.75 35.95,10.42 36.96,9.4 40.14,9.4 40.5,9.76 U$15.4
PJ3
  Top 0.178: IC1.66 30.79,23.09 32.92,20.96 35.96,20.96 R22.2
PK0
  Top 0.178: IC1.89 21.48,31.25 22.1,31.88 25.66,31.88 26.42,32.64 27.94,32.64 28.33,33.02 30.87,33.02 JP8.9
PK1  (via drill 0.38)
  Top 0.178: IC1.88 21.98,31.25 22.23,31.5 25.79,31.5 26.55,32.26 28.07,32.26 28.45,32.64 32.9,32.64 v33.41,33.15
  Bottom 0.178: v33.41,33.15 33.02,32.77 SJ103.3
  Bottom 0.254: SJ103.3 33.02,32.01
PK2  (via drill 0.38)
  Top 0.178: IC1.87 22.48,28.7 v21.98,28.2
  Bottom 0.178: SJ102.3 36.33,30.99 36.07,30.74 32.64,30.74 32.39,30.99 30.87,30.99 30.23,30.36 23.88,30.36 21.98,28.45 v21.98,28.2
PK3  (via drill 0.38)
  Top 0.178: IC1.86 22.98,28.47 v22.99,28.2
  Bottom 0.178: SJ101.3 39.63,30.99 39.37,30.74 36.58,30.74 36.2,30.36 32.52,30.36 32.26,30.61 30.99,30.61 30.36,29.98 24.01,29.98 22.99,28.96 v22.99,28.2
PK4  (via drill 0.38)
  Top 0.178: IC1.85 23.48,28.73 23.75,28.45 23.75,27.56 v23.63,27.44 | v10.29,10.93 10.55,10.67 10.55,5.97 10.29,5.72 U$17.3
  Bottom 0.178: v23.63,27.44 23.25,27.44 21.98,26.17 21.98,25.15 19.31,22.48 17.02,22.48 15.5,20.96 15.5,18.67 15.37,18.55 14.61,18.55 12.7,16.64 12.7,12.7 11.31,11.31 10.67,11.31 v10.29,10.93
PK5  (via drill 0.38)
  Top 0.178: IC1.84 23.98,28.74 24.52,28.2 v24.52,27.82
  Bottom 0.178: v24.52,27.82 24.52,27.18 24.13,26.8 23.12,26.8 22.36,26.04 22.36,25.02 19.44,22.1 17.15,22.1 15.88,20.83 15.88,18.55 15.5,18.17 14.74,18.17 13.09,16.51 13.09,12.58 10.67,10.16 8.13,10.16 7.62,9.66 5.47,9.66 5.08,9.28 5.08,5.97 5.72,5.34 7.37,5.34 8.26,4.45 9.27,4.45 U$17.4
PL1
  Top 0.178: IC1.36 20.98,12.69 21.09,12.58 23.37,12.58 24.52,11.43 R11.1
PL4  (via drill 0.38)
  Top 0.178: IC1.39 22.48,16.89 v22.48,17.02 | R21.1 35.45,29.83 35.18,30.1 34.29,30.1 v33.91,29.72
  Top 0.254: IC1.39
  Route15 0.178: v22.48,17.02 22.48,21.59 25.91,25.02 28.96,25.02 32.39,28.45 33.28,28.45 33.91,29.09 v33.91,29.72
PL5  (via drill 0.38)
  Top 0.178: IC1.40 22.98,15.99 v23.37,16.39 | v38.23,29.47 37.72,29.85 R24.1
  Route15 0.178: v23.37,16.39 23.37,17.4 22.86,17.91 22.86,21.47 26.04,24.64 29.09,24.64 32.52,28.07 36.07,28.07 36.33,28.33 36.33,29.21 36.58,29.47 v38.23,29.47
PPM_IN  (via drill 0.38)
  Top 0.178: v28.83,6.74 28.45,7.12 24.9,7.12 24.52,7.5 R11.2 24.5,9.53 23.25,9.53 22.86,9.91 TP2.TP
  Bottom 0.178: v28.83,6.74 29.47,7.37 31.88,7.37 33.02,8.51 43.95,8.51 44.33,8.89 50.68,8.89 53.73,11.94 53.73,16.77 53.22,17.28 SJ2.2
PPM_MISO  (via drill 0.38)
  Top 0.178: U10.17 55.48,23.65 v55.76,23.37 56.27,22.86 R42.2
  Bottom 0.178: U8.1 47.38,6.99 48.52,8.13 50.93,8.13 54.49,11.69 54.49,15.63 54.87,16.01 54.87,22.48 v55.76,23.37
PPM_MOSI  (via drill 0.38)
  Top 0.178: U10.16 54.21,22.64 54.74,22.1 55.5,22.1 v55.63,21.98 56.01,21.59 R43.2
  Bottom 0.178: U8.4 49.92,3.94 48.65,5.21 48.65,7.37 49.03,7.75 51.06,7.75 54.87,11.56 54.87,15.5 55.25,15.88 55.25,21.59 v55.63,21.98
PPM_OUT  (via drill 0.38)
  Top 0.178: U10.23 55.23,26.65 55.38,26.8 55.38,27.82 55.5,27.94 55.5,28.58 55.76,28.83 55.76,29.6 v55.12,30.23
  Bottom 0.178: v55.12,30.23 54.74,30.61 53.6,30.61 53.09,30.1 53.09,27.69 53.47,27.31 54.23,27.31 54.49,27.06 54.49,23.88 54.11,23.5 54.11,19.05 53.85,18.8 SJ2.1 51.69,17.4
PPM_PC2  (via drill 0.38)
  Top 0.178: U$7.1 34.41,26.69 v35.18,25.91 | U$7.5 32.41,26.82 32.39,26.8 v32.39,25.91 | U10.5 49.66,25.15 49.53,25.28 48.65,25.28 48.26,24.9 48.26,22.99 v48.42,22.89
  Route15 0.178: v48.42,22.89 47.88,22.36 47.25,22.36 46.11,23.5 45.09,23.5 43.06,25.53 37.72,25.53 37.6,25.4 35.69,25.4 v35.18,25.91
  Bottom 0.178: v35.18,25.91 35.06,25.79 35.06,25.4 34.8,25.15 33.66,25.15 33.15,25.66 32.64,25.66 v32.39,25.91
PPM_PC4  (via drill 0.38)
  Top 0.178: U10.26 53.71,28.43 v53.85,28.58 | v53.34,20.2 53.22,20.07 53.22,17.91 54.36,16.77 54.36,16.13 54.87,15.63 54.87,13.59 55.12,13.34 57.03,13.34 57.41,12.96 57.41,12.32 57.54,12.2 61.47,12.2 61.98,12.7 X4.1
  Route15 0.178: v53.85,28.58 53.85,21.85 54.11,21.59 54.11,20.96 v53.34,20.2
PPM_PD0  (via drill 0.38)
  Top 0.178: U10.6 49.17,24.65 v49.03,24.52 | 31.5,31.75 R47.2 31.12,31.75 30.87,31.5 30.87,29.47 v30.74,29.34
  Route15 0.178: v49.03,24.52 48.39,24.52 48.26,24.64 45.47,24.64 43.69,26.42 43.69,30.61 42.68,31.63 32.64,31.63 31.63,30.61 31.12,30.61 30.74,30.23 v30.74,29.34
PPM_PD1  (via drill 0.38)
  Top 0.178: U10.7 49.81,24.15 49.23,23.58 v49.23,23.37 | R46.2 31.52,29.99 v31.5,29.98
  Route15 0.178: v49.23,23.37 49.03,23.37 48.14,24.26 45.34,24.26 43.31,26.29 43.31,30.48 42.55,31.25 32.77,31.25 v31.5,29.98
PPM_PD6
  Top 0.178: U10.12 52.21,21.97 52.58,21.59 52.58,19.82 52.84,19.56 52.84,17.78 53.98,16.64 53.98,16.01 54.49,15.5 54.49,13.34 54.87,12.96 56.77,12.96 57.03,12.7 57.03,12.07 57.28,11.82 61.35,11.82 62.49,10.67 X2.1
PPM_RST  (via drill 0.38)
  Top 0.178: U10.24 54.76,27.83 55.12,28.2 v55.12,29.24 | R37.1 56.27,17.53 55.63,18.17 v54.11,18.17
  Bottom 0.178: U8.5 47.38,1.91 46.11,3.18 46.11,7.5 47.12,8.51 50.8,8.51 54.11,11.82 54.11,15.75 54.49,16.13 54.49,17.78 v54.11,18.17 54.49,18.55 54.49,23.37 54.87,23.75 54.87,27.06 55.12,27.31 v55.12,29.24
PPM_RX  (via drill 0.38)
  Top 0.178: U$7.4 32.91,29.86 33.53,30.48 38.74,30.48 39.63,29.6 40.64,29.6 v41.28,28.96 | U10.8 50.16,22.98 49.28,22.1 48.14,22.1 47.5,22.74 v47.5,23.12
  Route15 0.178: v47.5,23.12 46.74,23.88 45.22,23.88 42.93,26.17 42.93,28.83 42.8,28.96 v41.28,28.96
PPM_SCK  (via drill 0.38)
  Top 0.178: R44.2 56.76,20.45 v56.01,20.45 55.88,20.45 53.71,22.63 U10.15
  Bottom 0.178: U8.3 47.5,3.81 48.77,2.54 50.42,2.54 51.19,3.31 51.19,7.37 55.25,11.43 55.25,15.37 55.63,15.75 55.63,20.07 v56.01,20.45
PPM_TX  (via drill 0.38)
  Top 0.178: U$7.2 v33.91,25.9 v33.91,25.91 | U10.9 50.71,22.38 v50.42,22.1
  Route15 0.178: v50.42,22.1 50.3,22.23 48.26,22.23 48.01,21.98 47.12,21.98 45.98,23.12 44.96,23.12 42.93,25.15 37.85,25.15 37.72,25.02 34.8,25.02 v33.91,25.91
R_JP_RX
  Top 0.178: R49.1 11.82,32.52 11.31,33.02 10.55,33.02 10.16,33.41 10.16,35.31 9.02,36.45 U$20.3
R_JP_TX
  Top 0.178: R50.1 10.53,32.4 9.78,33.15 9.78,34.55 9.15,35.18 8.03,35.18 U$20.2
RD+
  Top 0.178: U10.29 52.21,31.25 52.71,31.75 52.71,32.26 52.47,32.37 R34.1
RD-
  Top 0.178: U10.30 51.71,31.26 51.19,31.75 R31.1
RST  (via drill 0.38)
  Top 0.178: v19.05,18.67 19.31,18.42 19.31,17.4 17.66,15.75 17.66,14.99 17.98,14.67 IC1.30 17.98,12.77 17.28,12.2 | C15.2 22.61,6.35 S1.3 | JP11.1 24.52,2.04 23.37,3.18 21.98,3.18 S1.3 | D3.A 17.28,6.35 19.18,4.45 S1.3
  Top 0.254: D2.C 42.23,32.33 R26.1 U7.5 | 17.28,12.2 17.28,10.42 17.66,10.04 18.8,10.04 19.31,9.53 19.31,8.01 18.8,7.5 17.46,7.5 D3.A
  Bottom 0.178: U7.5 43.18,33.41 43.18,28.58 42.42,27.82 40.9,27.82 39.88,26.8 38.49,26.8 37.85,27.44 31.5,27.44 29.09,25.02 25.4,25.02 v19.05,18.67
RST_DF
  Top 0.178: U$15.10 43.58,10.56 44.07,11.05 44.07,11.69 45.72,13.34 46.61,13.34 46.74,13.47 IC2.3
RXLED
  Top 0.178: U10.10 51.21,22.59 51.31,22.48 51.31,21.85 51.82,21.34 51.82,19.56 52.07,19.31 52.07,17.53 53.22,16.39 53.22,15.49 LED4.C
SCK_3V3
  Top 0.178: U5.23 43.58,21.07 44.33,20.32 45.17,20.32 | 45.17,20.32 46.6,20.32 U$12.8 | 45.17,20.32 45.17,21.77 44.96,21.98 44.96,22.86 44.58,23.25 40.01,23.25 39.36,23.9 U$14.2
SCK_DF
  Top 0.178: U$15.8 43.8,9.76 44.84,10.8 44.84,11.43 45.98,12.58 47.38,12.58 48.01,13.21 IC2.2
SCL1  (via drill 0.38)
  Top 0.178: v32.14,10.16 31.88,9.91 31.75,9.91 U2.2 | U$13.1 35.68,4.33 v35.69,4.32 | R9.1 13.22,4.58 U$19.2
  Route15 0.178: v35.69,4.32 35.82,4.32 36.58,5.08 36.58,6.99 36.2,7.37 35.31,7.37 32.77,9.91 32.39,9.91 v32.14,10.16
  Bottom 0.178: v32.14,10.16 32.01,10.16 29.98,8.13 28.33,8.13 27.31,7.12 15.5,7.12 14.99,6.61 14.99,4.96 14.48,4.45 U$19.2
SDA1  (via drill 0.38)
  Top 0.178: v29.72,6.48 29.72,7.88 30.48,8.64 | v31.63,8.64 30.48,8.64 | 30.48,8.64 30.23,8.89 30.23,10.16 30.48,10.41 U2.3 31.5,10.41 31.63,10.55 31.63,10.67 31.75,10.8 32.9,10.8 SJ6.2 | 13.08,3.18 U$19.3 13.2,3.31 R16.1
  Top 0.254: U2.3
  Bottom 0.178: v29.72,6.48 28.58,5.34 27.18,5.34 25.79,6.74 15.63,6.74 15.37,6.48 15.37,3.69 14.86,3.18 13.1,3.18 U$19.3
SJ0
  Bottom 0.178: SJ103.2 33.91,32.39 34.68,33.15 JP8.10
SJ1
  Bottom 0.178: SJ102.2 JP8.11
SJ2
  Bottom 0.178: SJ101.2 40.52,33.53 JP8.12
SPI_OE  (via drill 0.38)
  Top 0.178: R25.2 37.22,13.97 36.71,14.48 v36.71,14.99 | U$14.12 37.98,25.4 v37.22,26.04 | U$15.12 42.3,11.43 43.06,12.2 v43.06,12.83
  Top 0.203: D2.A 39.81,28.63 v39.12,27.94
  Route15 0.178: 36.71,27.69 32.64,27.69 30.1,25.15 30.1,22.23 31.37,20.96 33.79,20.96 35.18,19.56 35.18,17.15 36.71,15.63 v36.71,14.99 37.6,14.1 42.3,14.1 43.06,13.34 v43.06,12.83 | 36.71,27.69 38.87,27.69 v39.12,27.94 | v37.22,26.04 37.22,27.18 36.71,27.69
SS_3V3  (via drill 0.38)
  Top 0.178: U5.8 39.87,21.07 v40.03,21.21 | U$14.4 40.16,24.24 40.39,24.01 41.03,24.01 v41.41,24.39
  Bottom 0.178: v40.03,21.21 40.01,21.21 41.15,22.36 41.15,24.13 v41.41,24.39
TXLED
  Top 0.178: U10.11 51.71,21.96 52.2,21.47 52.2,19.69 52.46,19.44 52.46,17.66 53.6,16.51 53.6,15.37 53.73,15.24 LED5.C
USHIELD
  Top 0.178: L1.2 48.65,33.66
  Top 0.254: 48.65,33.66 49.53,32.77 49.79,32.77 49.92,32.64 Z1.2 | 56.65,39.03 U9.GND1 54.74,38.56 | 54.74,38.56 U9.GND2 U9.GND3 50.17,38.56 | 50.17,38.56 U9.GND4 | 50.17,38.56 50.17,37.34 49.92,37.09 48.9,37.09 48.52,36.83 48.52,35.18 48.65,35.06 L1.2 | 54.74,38.56 54.74,37.6 57.28,35.06 57.28,34.31 Z2.2
VCC  (via drill 0.38, 0.6)
  Top 0.178: U10.32 50.03,27.7 v49.53,28.2 49.55,28.2 R51.1 50.57,28.95 51.21,28.31 U10.31 | R14.1 31.52,19.05 C3.1 31.5,19.07 31.5,20.07 30.98,20.59 IC1.61 26.56,20.59 v26.29,20.32 | IC1.80 25.98,28.64 v26.42,28.2 | IC1.31 18.48,15.32 v18.42,15.37 | IC1.10 15.73,23.09 v16.39,23.75 | C5.2 35.82,23.37 | U$7.8 33.41,22.36 33.79,21.98 36.58,21.98 v36.96,22.36 | R32.1 R35.1 R36.2 55,10.29 55.5,9.78 58.3,9.78 58.81,9.28 58.81,8.05 U$18.1 | U10.25 54.21,27.92 54.49,28.2 54.49,28.96 v53.85,29.6 | C14.1 46.34,23.75 47.25,23.75 47.88,24.39 47.88,25.02 48.51,25.65 48.87,25.65 v49.23,26.01 49.59,25.65 U10.4 | U$14.11 38.96,26.46 38.61,26.8 36.96,26.8 36.58,26.42 36.58,25.53 37.47,24.64 37.47,23.75 36.96,23.25 | R26.2 42.3,30.61 v41.66,29.98 | v58.42,14.23 57.54,15.12 C16.1 R37.2 | D3.C 19.82,6.35 | C2.1 13.48,28.96 v15.12,28.96 15.75,29.59 IC1.100 | U$15.11 43.48,10.96 43.69,11.18 43.69,11.82 44.2,12.32 v44.2,13.09
  Top 0.254: IC1.100 | R12.2 26.56,9.51 v27.18,8.89 | v36.96,22.36 36.96,23.25 36.72,23.48 35.83,23.48 | F1.2 58.81,39.25 60.46,37.6 60.46,36.45 JP18.1 | R20.2 R18.2 R13.2 1.01,5.32 v0.89,5.21 | GPS.5 57.77,6.33 58.68,7.24 58.68,7.92 U$18.1 | v20.45,5.59 20.45,5.92 D3.C
  Top 0.305: 35.83,23.48 C5.2 | JP14.3 38.49,2.67 37.22,2.67 36.83,3.05 36.83,3.81 | 36.83,3.81 36.83,4.7 37.23,5.1 U$3.1 37.59,6.74 C6.2 | U$3.3 36.85,3.8 36.83,3.81
  Top 0.61: F2.2 16.26,8.95 D4.C v17.28,8.89
  other vias: 16.26,9.91
  pour Route2 (isolate 0.254): 0,40.64 68.97,40.64 68.97,0 0,0
VUCAP
  Top 0.178: U10.27 53.21,28.08 52.58,28.71 52.58,30.87 52.84,31.12 53.71,31.12 C17.1
XT1
  Top 0.178: R28.1 R29.2 46.73,27.02 Y1.3
XT1R
  Top 0.178: U10.1 49.56,27.15 48.77,27.94 48.77,28.47 R28.2
XT2
  Top 0.178: Y1.1 47.39,24.66 47.5,24.77 47.5,25.28 48.65,26.42 48.65,27.08 48.89,27.32 | U10.2 49.66,26.65 49.53,26.78 49.43,26.78 48.89,27.32 | 48.89,27.32 48.52,27.69 48.28,27.69 R29.1
XUSB
  Top 0.254: U9.1 53.76,33.88 54.23,33.41 58.17,33.41 58.42,33.66 58.42,35.31 58.81,35.69 F1.1

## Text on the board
tPlace: 3DR-RADIO | + | - | AREF | AT2560 SPI | OUT | - | + | s | Inputs | Outputs | JP | 1 | Front | s | JP4 | + | - | TX | RX | Alive | JP3 | PPM | GPS/UART1 | JP2 | C | B | I2C | ATx-U2 | A | Reset | PM
bPlace: MISO LVL | GND | UART0/2 | RX | TX | 5V | 3V3 | IN8 | +5V | A0 | A1 | A2 | A3 | A4 | A5 | A6 | A7 | A8 | IN7 | UART2 | UART0 | A9 | OUT9 | A10 | OUT10 | A11 | OUT11 | IN6 | OUT8 | Inputs | IN5 | OUT7 | AutoMUX | IN4 | OUT6 | FRONT | IN3 | OUT5 | OUT4 | <-PPM | IN2 | ->PPM | Outputs | IN1 | OUT3 | <-CH5 | OUT2 | S | JP4 | + | - | JP1 | JP3 | OUT1 | GPS/UART1 | - | 5V | S | JP2 | V2.5 | RESET | UART2 | UART0 | PWR-M&R | I2C | GND | 3v3 | GND | RST | GND | +5V | RX2 | TX2 | GND | +5V | TX0 | RX0
tNames: 3D Robotics Inc.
